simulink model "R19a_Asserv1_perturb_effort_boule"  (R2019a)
settings: Solver=ode15s  StartTime=0.0  StopTime=1  RelTol=1e-3  EnableMultiTasking=on
undefined symbols (not defined in the file): deg, kg, m, manette1_Défaut_sldprt, manette2_Défaut_sldprt, mm, N, rad, s, sigbuilder_block, STL, X, Y, Z
libraries: sm_lib x460, fl_lib x45, nesl_utility x23, simulink x3
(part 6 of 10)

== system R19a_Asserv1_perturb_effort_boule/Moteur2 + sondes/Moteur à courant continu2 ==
  note: Kv = 1.18e-1
  Frottement : fl_lib/Mechanical/Rotational Elements/Rotational Friction  brkwy_trq=2.43e-3 N*m  brkwy_vel=0.030296 rad/s  Col_trq=2.43e-3 N*m  visc_coef=2e-6 N*m/(rad/s)  w_specify=off  w_priority=High  w=0 rad/s  w_nominal_specify=off  w_nominal_unit=rad/s  w_nominal_value=1  t_specify=off  t_priority=High  t=0 N*m  t_nominal_specify=off  t_nominal_unit=N*m  t_nominal_value=1
  Inductance induit 35mH : fl_lib/Electrical/Electrical Elements/Inductor  l=35 mH  r=0 Ohm  g=1e-09 1/Ohm  i_specify=off  i_priority=High  i=0 A  i_nominal_specify=off  i_nominal_unit=A  i_nominal_value=1  v_specify=off  v_priority=High  v=0 V  v_nominal_specify=off  v_nominal_unit=V  v_nominal_value=1  i_L_specify=on  i_L_priority=High  i_L=0 A  i_L_nominal_specify=off  i_L_nominal_unit=A  i_L_nominal_value=1
  Inertie Je 10e-6 : fl_lib/Mechanical/Rotational Elements/Inertia  inertia=10.5e-6 kg*m^2  w_specify=on  w_priority=High  w=0 rad/s  w_nominal_specify=off  w_nominal_unit=rad/s  w_nominal_value=1  t_specify=off  t_priority=High  t=0 N*m  t_nominal_specify=off  t_nominal_unit=N*m  t_nominal_value=1
  Moteur parfait : fl_lib/Electrical/Electrical Elements/Rotational Electromechanical Converter  K=1.18e-1 V/(rad/s)  i_specify=off  i_priority=High  i=0 A  i_nominal_specify=off  i_nominal_unit=A  i_nominal_value=1  v_specify=off  v_priority=High  v=0 V  v_nominal_specify=off  v_nominal_unit=V  v_nominal_value=1  t_specify=off  t_priority=High  t=0 N*m  t_nominal_specify=off  t_nominal_unit=N*m  t_nominal_value=1  w_specify=off  w_priority=High  w=0 rad/s  w_nominal_specify=off  w_nominal_unit=rad/s  w_nominal_value=1
  Rinduit 38 Ohms : fl_lib/Electrical/Electrical Elements/Resistor  Tag=Factory Generic  R=38 Ohm  i_specify=off  i_priority=High  i=0 A  i_nominal_specify=off  i_nominal_unit=A  i_nominal_value=1  v_specify=off  v_priority=High  v=0 V  v_nominal_specify=off  v_nominal_unit=V  v_nominal_value=1
  V+ : PMIOPort  Side=Left
  R : PMIOPort  Port=2  Side=Right
  C : PMIOPort  Port=3  Side=Right
  V- : PMIOPort  Port=4  Side=Left
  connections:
  Moteur parfait/LConn1 -- Inductance induit 35mH/RConn1
  V-/RConn1 -- Moteur parfait/RConn1
  Rinduit 38 Ohms/LConn1 -- V+/RConn1
  Inductance induit 35mH/LConn1 -- Rinduit 38 Ohms/RConn1
  Frottement/LConn1 -- Moteur parfait/LConn2 -- Inertie Je 10e-6/LConn1 -- R/RConn1
  Frottement/RConn1 -- Moteur parfait/RConn2 -- C/RConn1

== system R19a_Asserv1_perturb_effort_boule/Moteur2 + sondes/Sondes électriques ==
  " Conv i" : nesl_utility/PS-Simulink Converter  PhysicalDomain=network_engine_domain  SubClassName=ps_output  LeftPortType=input  RightPortType=output  PseudoPeriodic=off  Frequencies=[]  Unit=1  AffineConversion=off
  " Conv v" : nesl_utility/PS-Simulink Converter  PhysicalDomain=network_engine_domain  SubClassName=ps_output  LeftPortType=input  RightPortType=output  PseudoPeriodic=off  Frequencies=[]  Unit=1  AffineConversion=off
  Bras2 : Scope  NumInputPorts=2
  Sonde_I : fl_lib/Electrical/Electrical Sensors/Current Sensor
  Sonde_U : fl_lib/Electrical/Electrical Sensors/Voltage Sensor
  Conn1 : PMIOPort  Side=Left
  Conn2 : PMIOPort  Port=2  Side=Right
  Conn3 : PMIOPort  Port=3  Side=Right
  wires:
  " Conv v"/1 -> [u]
  " Conv i"/1 -> [i]
  [u] -> Bras2/1  "Umoteur2"
  [i] -> Bras2/2  "Imoteur2"
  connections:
  Sonde_I/RConn1 -- " Conv i"/LConn1
  Sonde_U/RConn1 -- " Conv v"/LConn1
  Conn1/RConn1 -- Sonde_U/LConn1 -- Sonde_I/LConn1
  Conn2/RConn1 -- Sonde_I/RConn2
  Conn3/RConn1 -- Sonde_U/RConn2

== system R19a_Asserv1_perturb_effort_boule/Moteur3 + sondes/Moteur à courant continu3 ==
  note: Kv = 1.18e-1
  Frottement : fl_lib/Mechanical/Rotational Elements/Rotational Friction  brkwy_trq=2.43e-3 N*m  brkwy_vel=0.030296 rad/s  Col_trq=2.43e-3 N*m  visc_coef=2e-6 N*m/(rad/s)  w_specify=off  w_priority=High  w=0 rad/s  w_nominal_specify=off  w_nominal_unit=rad/s  w_nominal_value=1  t_specify=off  t_priority=High  t=0 N*m  t_nominal_specify=off  t_nominal_unit=N*m  t_nominal_value=1
  Inductance induit 35mH : fl_lib/Electrical/Electrical Elements/Inductor  l=35 mH  r=0 Ohm  g=1e-09 1/Ohm  i_specify=off  i_priority=High  i=0 A  i_nominal_specify=off  i_nominal_unit=A  i_nominal_value=1  v_specify=off  v_priority=High  v=0 V  v_nominal_specify=off  v_nominal_unit=V  v_nominal_value=1  i_L_specify=on  i_L_priority=High  i_L=0 A  i_L_nominal_specify=off  i_L_nominal_unit=A  i_L_nominal_value=1
  Inertie Je 10e-6 : fl_lib/Mechanical/Rotational Elements/Inertia  inertia=10.5e-6 kg*m^2  w_specify=on  w_priority=High  w=0 rad/s  w_nominal_specify=off  w_nominal_unit=rad/s  w_nominal_value=1  t_specify=off  t_priority=High  t=0 N*m  t_nominal_specify=off  t_nominal_unit=N*m  t_nominal_value=1
  Moteur parfait : fl_lib/Electrical/Electrical Elements/Rotational Electromechanical Converter  K=1.18e-1 V/(rad/s)  i_specify=off  i_priority=High  i=0 A  i_nominal_specify=off  i_nominal_unit=A  i_nominal_value=1  v_specify=off  v_priority=High  v=0 V  v_nominal_specify=off  v_nominal_unit=V  v_nominal_value=1  t_specify=off  t_priority=High  t=0 N*m  t_nominal_specify=off  t_nominal_unit=N*m  t_nominal_value=1  w_specify=off  w_priority=High  w=0 rad/s  w_nominal_specify=off  w_nominal_unit=rad/s  w_nominal_value=1
  Rinduit 38 Ohms : fl_lib/Electrical/Electrical Elements/Resistor  Tag=Factory Generic  R=38 Ohm  i_specify=off  i_priority=High  i=0 A  i_nominal_specify=off  i_nominal_unit=A  i_nominal_value=1  v_specify=off  v_priority=High  v=0 V  v_nominal_specify=off  v_nominal_unit=V  v_nominal_value=1
  V+ : PMIOPort  Side=Left
  R : PMIOPort  Port=2  Side=Right
  C : PMIOPort  Port=3  Side=Right
  V- : PMIOPort  Port=4  Side=Left
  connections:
  Moteur parfait/LConn1 -- Inductance induit 35mH/RConn1
  V-/RConn1 -- Moteur parfait/RConn1
  Rinduit 38 Ohms/LConn1 -- V+/RConn1
  Inductance induit 35mH/LConn1 -- Rinduit 38 Ohms/RConn1
  Frottement/LConn1 -- Moteur parfait/LConn2 -- Inertie Je 10e-6/LConn1 -- R/RConn1
  Frottement/RConn1 -- Moteur parfait/RConn2 -- C/RConn1

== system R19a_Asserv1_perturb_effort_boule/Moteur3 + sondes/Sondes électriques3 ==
  " Conv i" : nesl_utility/PS-Simulink Converter  PhysicalDomain=network_engine_domain  SubClassName=ps_output  LeftPortType=input  RightPortType=output  PseudoPeriodic=off  Frequencies=[]  Unit=1  AffineConversion=off
  " Conv v" : nesl_utility/PS-Simulink Converter  PhysicalDomain=network_engine_domain  SubClassName=ps_output  LeftPortType=input  RightPortType=output  PseudoPeriodic=off  Frequencies=[]  Unit=1  AffineConversion=off
  Bras3 : Scope  NumInputPorts=2
  Sonde_I : fl_lib/Electrical/Electrical Sensors/Current Sensor
  Sonde_U : fl_lib/Electrical/Electrical Sensors/Voltage Sensor
  Conn1 : PMIOPort  Side=Left
  Conn2 : PMIOPort  Port=2  Side=Right
  Conn3 : PMIOPort  Port=3  Side=Right
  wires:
  " Conv v"/1 -> [u]
  " Conv i"/1 -> [i]
  [u] -> Bras3/1  "Umoteur3"
  [i] -> Bras3/2  "Imoteur3"
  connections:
  Sonde_I/RConn1 -- " Conv i"/LConn1
  Sonde_U/RConn1 -- " Conv v"/LConn1
  Conn1/RConn1 -- Sonde_U/LConn1 -- Sonde_I/LConn1
  Conn2/RConn1 -- Sonde_I/RConn2
  Conn3/RConn1 -- Sonde_U/RConn2

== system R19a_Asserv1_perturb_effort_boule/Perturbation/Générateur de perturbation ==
  Demux : Demux  Tag=STV Demux  Outputs=1
  FromWs : FromWorkspace  Tag=STV FromWs  VariableName=tuvar  SampleTime=0
  Signal 1 : Outport  Tag=STV Outport
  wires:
  Demux/1 -> Signal 1/1
  FromWs/1 -> Demux/1

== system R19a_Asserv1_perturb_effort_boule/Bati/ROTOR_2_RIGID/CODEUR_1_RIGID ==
  ReferenceFrame : sm_lib/Frames and Transforms/Reference Frame
  Solid : sm_lib/Body Elements/Solid  InertiaType=Custom  Mass=0.0064318274490095598  MassUnits=kg  CenterOfMass=[0 6.0527709306807029 -0.1964144966449296]  CenterOfMassUnits=mm  MomentsOfInertia=[0.92812714377460337 1.2443807481520079 0.93469179577802664]  MomentsOfInertiaUnits=kg*mm^2  ProductsOfInertia=[0.0063987198741970201 0 0]  ProductsOfInertiaUnits=kg*mm^2  BasedOnType=Density  Density=1000  DensityUnits=kg/(m^3)  DoExposeReferenceFrame=on  SerializedFrames=<Frames/>  GraphicType=FromGeometry  MarkerShape=Sphere  MarkerSize=10  MarkerSizeUnits=m  GraphicVisPropType=SimpleVisualProperties  GraphicDiffuseColor=[0.2 1.0 0.2]  GraphicSpecularColor=[0.5 0.5 0.5 1.0]  GraphicAmbientColor=[0.15 0.15 0.15 1.0]  GraphicEmissiveColor=[0.0 0.0 0.0 1.0]  GraphicShininess=75  GraphicOpacity=1  GeometryShape=FromFile  RectangleSize=[1 1]  RectangleSizeUnits=m  BrickDimensions=[1 1 1]  BrickDimensionUnits=m  CylinderRadius=1  CylinderRadiusUnits=m  CylinderLength=1  CylinderLengthUnits=m  SphereRadius=1  SphereRadiusUnits=m  EllipsoidRadii=[1 1 1]  EllipsoidRadiiUnits=m  ExtrusionCrossSection=[1 1; -1 1; -1 -1; 1 -1]  ExtrusionCrossSectionUnits=m  ExtrusionLength=1  ExtrusionLengthUnits=m  PolygonNumSides=3  PolygonOuterRadius=1  PolygonOuterRadiusUnits=m  ExtGeomFileType=STL  ExtGeomFileName=\STL\CODEUR_Défaut_sldprt.STL  ExtGeomFileUnits=mm  RevolutionCrossSection=[1 1; 1 -1; 2 -1; 2 1]  RevolutionCrossSectionUnits=m  RevolutionExtent=Full  RevolutionAngle=180  RevolutionAngleUnits=deg
  F : PMIOPort  Side=Left
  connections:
  Solid/RConn1 -- ReferenceFrame/RConn1 -- F/RConn1

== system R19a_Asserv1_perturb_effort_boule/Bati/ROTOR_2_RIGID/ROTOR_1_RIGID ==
  ReferenceFrame : sm_lib/Frames and Transforms/Reference Frame
  Solid : sm_lib/Body Elements/Solid  InertiaType=Custom  Mass=0.07643998420030651  MassUnits=kg  CenterOfMass=[0 30.928341108151987 -0.0018262913863015125]  CenterOfMassUnits=mm  MomentsOfInertia=[14.640748377051393 9.6696912582654697 14.640902193857929]  MomentsOfInertiaUnits=kg*mm^2  ProductsOfInertia=[0.0065014820412302417 0 0]  ProductsOfInertiaUnits=kg*mm^2  BasedOnType=Density  Density=1000  DensityUnits=kg/(m^3)  DoExposeReferenceFrame=on  SerializedFrames=<Frames/>  GraphicType=FromGeometry  MarkerShape=Sphere  MarkerSize=10  MarkerSizeUnits=m  GraphicVisPropType=SimpleVisualProperties  GraphicDiffuseColor=[0.53725490196078429 0.34901960784313724 0.33725490196078434]  GraphicSpecularColor=[0.5 0.5 0.5 1.0]  GraphicAmbientColor=[0.15 0.15 0.15 1.0]  GraphicEmissiveColor=[0.0 0.0 0.0 1.0]  GraphicShininess=75  GraphicOpacity=1  GeometryShape=FromFile  RectangleSize=[1 1]  RectangleSizeUnits=m  BrickDimensions=[1 1 1]  BrickDimensionUnits=m  CylinderRadius=1  CylinderRadiusUnits=m  CylinderLength=1  CylinderLengthUnits=m  SphereRadius=1  SphereRadiusUnits=m  EllipsoidRadii=[1 1 1]  EllipsoidRadiiUnits=m  ExtrusionCrossSection=[1 1; -1 1; -1 -1; 1 -1]  ExtrusionCrossSectionUnits=m  ExtrusionLength=1  ExtrusionLengthUnits=m  PolygonNumSides=3  PolygonOuterRadius=1  PolygonOuterRadiusUnits=m  ExtGeomFileType=STL  ExtGeomFileName=\STL\ROTOR_Défaut_sldprt.STL  ExtGeomFileUnits=mm  RevolutionCrossSection=[1 1; 1 -1; 2 -1; 2 1]  RevolutionCrossSectionUnits=m  RevolutionExtent=Full  RevolutionAngle=180  RevolutionAngleUnits=deg
  F : PMIOPort  Side=Left
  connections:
  Solid/RConn1 -- ReferenceFrame/RConn1 -- F/RConn1

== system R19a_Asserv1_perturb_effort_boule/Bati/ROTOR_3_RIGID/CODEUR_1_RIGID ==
  ReferenceFrame : sm_lib/Frames and Transforms/Reference Frame
  Solid : sm_lib/Body Elements/Solid  InertiaType=Custom  Mass=0.0064318274490095598  MassUnits=kg  CenterOfMass=[0 6.0527709306807029 -0.1964144966449296]  CenterOfMassUnits=mm  MomentsOfInertia=[0.92812714377460337 1.2443807481520079 0.93469179577802664]  MomentsOfInertiaUnits=kg*mm^2  ProductsOfInertia=[0.0063987198741970201 0 0]  ProductsOfInertiaUnits=kg*mm^2  BasedOnType=Density  Density=1000  DensityUnits=kg/(m^3)  DoExposeReferenceFrame=on  SerializedFrames=<Frames/>  GraphicType=FromGeometry  MarkerShape=Sphere  MarkerSize=10  MarkerSizeUnits=m  GraphicVisPropType=SimpleVisualProperties  GraphicDiffuseColor=[0.792156862745098 0.81960784313725488 0.93333333333333335]  GraphicSpecularColor=[0.5 0.5 0.5 1.0]  GraphicAmbientColor=[0.15 0.15 0.15 1.0]  GraphicEmissiveColor=[0.0 0.0 0.0 1.0]  GraphicShininess=75  GraphicOpacity=1  GeometryShape=FromFile  RectangleSize=[1 1]  RectangleSizeUnits=m  BrickDimensions=[1 1 1]  BrickDimensionUnits=m  CylinderRadius=1  CylinderRadiusUnits=m  CylinderLength=1  CylinderLengthUnits=m  SphereRadius=1  SphereRadiusUnits=m  EllipsoidRadii=[1 1 1]  EllipsoidRadiiUnits=m  ExtrusionCrossSection=[1 1; -1 1; -1 -1; 1 -1]  ExtrusionCrossSectionUnits=m  ExtrusionLength=1  ExtrusionLengthUnits=m  PolygonNumSides=3  PolygonOuterRadius=1  PolygonOuterRadiusUnits=m  ExtGeomFileType=STL  ExtGeomFileName=\STL\CODEUR_Défaut_sldprt.STL  ExtGeomFileUnits=mm  RevolutionCrossSection=[1 1; 1 -1; 2 -1; 2 1]  RevolutionCrossSectionUnits=m  RevolutionExtent=Full  RevolutionAngle=180  RevolutionAngleUnits=deg
  F : PMIOPort  Side=Left
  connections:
  Solid/RConn1 -- ReferenceFrame/RConn1 -- F/RConn1

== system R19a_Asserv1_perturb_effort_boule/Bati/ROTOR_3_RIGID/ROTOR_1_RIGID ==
  ReferenceFrame : sm_lib/Frames and Transforms/Reference Frame
  Solid : sm_lib/Body Elements/Solid  InertiaType=Custom  Mass=0.07643998420030651  MassUnits=kg  CenterOfMass=[0 30.928341108151987 -0.0018262913863015125]  CenterOfMassUnits=mm  MomentsOfInertia=[14.640748377051393 9.6696912582654697 14.640902193857929]  MomentsOfInertiaUnits=kg*mm^2  ProductsOfInertia=[0.0065014820412302417 0 0]  ProductsOfInertiaUnits=kg*mm^2  BasedOnType=Density  Density=1000  DensityUnits=kg/(m^3)  DoExposeReferenceFrame=on  SerializedFrames=<Frames/>  GraphicType=FromGeometry  MarkerShape=Sphere  MarkerSize=10  MarkerSizeUnits=m  GraphicVisPropType=SimpleVisualProperties  GraphicDiffuseColor=[0.53725490196078429 0.34901960784313724 0.33725490196078434]  GraphicSpecularColor=[0.5 0.5 0.5 1.0]  GraphicAmbientColor=[0.15 0.15 0.15 1.0]  GraphicEmissiveColor=[0.0 0.0 0.0 1.0]  GraphicShininess=75  GraphicOpacity=1  GeometryShape=FromFile  RectangleSize=[1 1]  RectangleSizeUnits=m  BrickDimensions=[1 1 1]  BrickDimensionUnits=m  CylinderRadius=1  CylinderRadiusUnits=m  CylinderLength=1  CylinderLengthUnits=m  SphereRadius=1  SphereRadiusUnits=m  EllipsoidRadii=[1 1 1]  EllipsoidRadiiUnits=m  ExtrusionCrossSection=[1 1; -1 1; -1 -1; 1 -1]  ExtrusionCrossSectionUnits=m  ExtrusionLength=1  ExtrusionLengthUnits=m  PolygonNumSides=3  PolygonOuterRadius=1  PolygonOuterRadiusUnits=m  ExtGeomFileType=STL  ExtGeomFileName=\STL\ROTOR_Défaut_sldprt.STL  ExtGeomFileUnits=mm  RevolutionCrossSection=[1 1; 1 -1; 2 -1; 2 1]  RevolutionCrossSectionUnits=m  RevolutionExtent=Full  RevolutionAngle=180  RevolutionAngleUnits=deg
  F : PMIOPort  Side=Left
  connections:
  Solid/RConn1 -- ReferenceFrame/RConn1 -- F/RConn1

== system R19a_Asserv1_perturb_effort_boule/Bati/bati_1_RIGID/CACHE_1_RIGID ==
  ReferenceFrame : sm_lib/Frames and Transforms/Reference Frame
  Solid : sm_lib/Body Elements/Solid  InertiaType=Custom  Mass=0.011182198960412355  MassUnits=kg  CenterOfMass=[4.3076392714328797 208.54208665729635 7.8822671814956502]  CenterOfMassUnits=mm  MomentsOfInertia=[9.7659613803690544 11.857978985199471 3.5448360594417863]  MomentsOfInertiaUnits=kg*mm^2  ProductsOfInertia=[-0.087124917777044883 -0.069374532976861802 0.10473407202046144]  ProductsOfInertiaUnits=kg*mm^2  BasedOnType=Density  Density=1000  DensityUnits=kg/(m^3)  DoExposeReferenceFrame=on  SerializedFrames=<Frames/>  GraphicType=FromGeometry  MarkerShape=Sphere  MarkerSize=10  MarkerSizeUnits=m  GraphicVisPropType=SimpleVisualProperties  GraphicDiffuseColor=[0.75294117647058822 0.75294117647058822 0.75294117647058822]  GraphicSpecularColor=[0.5 0.5 0.5 1.0]  GraphicAmbientColor=[0.15 0.15 0.15 1.0]  GraphicEmissiveColor=[0.0 0.0 0.0 1.0]  GraphicShininess=75  GraphicOpacity=1  GeometryShape=FromFile  RectangleSize=[1 1]  RectangleSizeUnits=m  BrickDimensions=[1 1 1]  BrickDimensionUnits=m  CylinderRadius=1  CylinderRadiusUnits=m  CylinderLength=1  CylinderLengthUnits=m  SphereRadius=1  SphereRadiusUnits=m  EllipsoidRadii=[1 1 1]  EllipsoidRadiiUnits=m  ExtrusionCrossSection=[1 1; -1 1; -1 -1; 1 -1]  ExtrusionCrossSectionUnits=m  ExtrusionLength=1  ExtrusionLengthUnits=m  PolygonNumSides=3  PolygonOuterRadius=1  PolygonOuterRadiusUnits=m  ExtGeomFileType=STL  ExtGeomFileName=\STL\CACHE_Défaut_sldprt.STL  ExtGeomFileUnits=mm  RevolutionCrossSection=[1 1; 1 -1; 2 -1; 2 1]  RevolutionCrossSectionUnits=m  RevolutionExtent=Full  RevolutionAngle=180  RevolutionAngleUnits=deg
  F : PMIOPort  Side=Left
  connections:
  Solid/RConn1 -- ReferenceFrame/RConn1 -- F/RConn1

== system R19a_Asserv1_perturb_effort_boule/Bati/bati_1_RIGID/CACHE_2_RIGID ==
  ReferenceFrame : sm_lib/Frames and Transforms/Reference Frame
  Solid : sm_lib/Body Elements/Solid  InertiaType=Custom  Mass=0.011182198960412355  MassUnits=kg  CenterOfMass=[4.3076392714328797 208.54208665729635 7.8822671814956502]  CenterOfMassUnits=mm  MomentsOfInertia=[9.7659613803690544 11.857978985199471 3.5448360594417863]  MomentsOfInertiaUnits=kg*mm^2  ProductsOfInertia=[-0.087124917777044883 -0.069374532976861802 0.10473407202046144]  ProductsOfInertiaUnits=kg*mm^2  BasedOnType=Density  Density=1000  DensityUnits=kg/(m^3)  DoExposeReferenceFrame=on  SerializedFrames=<Frames/>  GraphicType=FromGeometry  MarkerShape=Sphere  MarkerSize=10  MarkerSizeUnits=m  GraphicVisPropType=SimpleVisualProperties  GraphicDiffuseColor=[0.75294117647058822 0.75294117647058822 0.75294117647058822]  GraphicSpecularColor=[0.5 0.5 0.5 1.0]  GraphicAmbientColor=[0.15 0.15 0.15 1.0]  GraphicEmissiveColor=[0.0 0.0 0.0 1.0]  GraphicShininess=75  GraphicOpacity=1  GeometryShape=FromFile  RectangleSize=[1 1]  RectangleSizeUnits=m  BrickDimensions=[1 1 1]  BrickDimensionUnits=m  CylinderRadius=1  CylinderRadiusUnits=m  CylinderLength=1  CylinderLengthUnits=m  SphereRadius=1  SphereRadiusUnits=m  EllipsoidRadii=[1 1 1]  EllipsoidRadiiUnits=m  ExtrusionCrossSection=[1 1; -1 1; -1 -1; 1 -1]  ExtrusionCrossSectionUnits=m  ExtrusionLength=1  ExtrusionLengthUnits=m  PolygonNumSides=3  PolygonOuterRadius=1  PolygonOuterRadiusUnits=m  ExtGeomFileType=STL  ExtGeomFileName=\STL\CACHE_Défaut_sldprt.STL  ExtGeomFileUnits=mm  RevolutionCrossSection=[1 1; 1 -1; 2 -1; 2 1]  RevolutionCrossSectionUnits=m  RevolutionExtent=Full  RevolutionAngle=180  RevolutionAngleUnits=deg
  F : PMIOPort  Side=Left
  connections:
  Solid/RConn1 -- ReferenceFrame/RConn1 -- F/RConn1

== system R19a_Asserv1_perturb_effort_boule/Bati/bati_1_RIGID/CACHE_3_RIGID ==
  ReferenceFrame : sm_lib/Frames and Transforms/Reference Frame
  Solid : sm_lib/Body Elements/Solid  InertiaType=Custom  Mass=0.011182198960412355  MassUnits=kg  CenterOfMass=[4.3076392714328797 208.54208665729635 7.8822671814956502]  CenterOfMassUnits=mm  MomentsOfInertia=[9.7659613803690544 11.857978985199471 3.5448360594417863]  MomentsOfInertiaUnits=kg*mm^2  ProductsOfInertia=[-0.087124917777044883 -0.069374532976861802 0.10473407202046144]  ProductsOfInertiaUnits=kg*mm^2  BasedOnType=Density  Density=1000  DensityUnits=kg/(m^3)  DoExposeReferenceFrame=on  SerializedFrames=<Frames/>  GraphicType=FromGeometry  MarkerShape=Sphere  MarkerSize=10  MarkerSizeUnits=m  GraphicVisPropType=SimpleVisualProperties  GraphicDiffuseColor=[0.75294117647058822 0.75294117647058822 0.75294117647058822]  GraphicSpecularColor=[0.5 0.5 0.5 1.0]  GraphicAmbientColor=[0.15 0.15 0.15 1.0]  GraphicEmissiveColor=[0.0 0.0 0.0 1.0]  GraphicShininess=75  GraphicOpacity=1  GeometryShape=FromFile  RectangleSize=[1 1]  RectangleSizeUnits=m  BrickDimensions=[1 1 1]  BrickDimensionUnits=m  CylinderRadius=1  CylinderRadiusUnits=m  CylinderLength=1  CylinderLengthUnits=m  SphereRadius=1  SphereRadiusUnits=m  EllipsoidRadii=[1 1 1]  EllipsoidRadiiUnits=m  ExtrusionCrossSection=[1 1; -1 1; -1 -1; 1 -1]  ExtrusionCrossSectionUnits=m  ExtrusionLength=1  ExtrusionLengthUnits=m  PolygonNumSides=3  PolygonOuterRadius=1  PolygonOuterRadiusUnits=m  ExtGeomFileType=STL  ExtGeomFileName=\STL\CACHE_Défaut_sldprt.STL  ExtGeomFileUnits=mm  RevolutionCrossSection=[1 1; 1 -1; 2 -1; 2 1]  RevolutionCrossSectionUnits=m  RevolutionExtent=Full  RevolutionAngle=180  RevolutionAngleUnits=deg
  F : PMIOPort  Side=Left
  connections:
  Solid/RConn1 -- ReferenceFrame/RConn1 -- F/RConn1

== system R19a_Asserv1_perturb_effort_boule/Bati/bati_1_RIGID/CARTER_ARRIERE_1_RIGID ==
  ReferenceFrame : sm_lib/Frames and Transforms/Reference Frame
  Solid : sm_lib/Body Elements/Solid  InertiaType=Custom  Mass=0.12081050845213158  MassUnits=kg  CenterOfMass=[0.027688933623677491 107.2258121438302 -1.1182869436416025]  CenterOfMassUnits=mm  MomentsOfInertia=[436.20873458136924 359.38976174708495 770.46596034318191]  MomentsOfInertiaUnits=kg*mm^2  ProductsOfInertia=[18.068269630416292 -0.016904145152124985 0.032703140147255623]  ProductsOfInertiaUnits=kg*mm^2  BasedOnType=Density  Density=1000  DensityUnits=kg/(m^3)  DoExposeReferenceFrame=on  SerializedFrames=<Frames/>  GraphicType=FromGeometry  MarkerShape=Sphere  MarkerSize=10  MarkerSizeUnits=m  GraphicVisPropType=SimpleVisualProperties  GraphicDiffuseColor=[1 1 1]  GraphicSpecularColor=[0.5 0.5 0.5 1.0]  GraphicAmbientColor=[0.15 0.15 0.15 1.0]  GraphicEmissiveColor=[0.0 0.0 0.0 1.0]  GraphicShininess=75  GraphicOpacity=1  GeometryShape=FromFile  RectangleSize=[1 1]  RectangleSizeUnits=m  BrickDimensions=[1 1 1]  BrickDimensionUnits=m  CylinderRadius=1  CylinderRadiusUnits=m  CylinderLength=1  CylinderLengthUnits=m  SphereRadius=1  SphereRadiusUnits=m  EllipsoidRadii=[1 1 1]  EllipsoidRadiiUnits=m  ExtrusionCrossSection=[1 1; -1 1; -1 -1; 1 -1]  ExtrusionCrossSectionUnits=m  ExtrusionLength=1  ExtrusionLengthUnits=m  PolygonNumSides=3  PolygonOuterRadius=1  PolygonOuterRadiusUnits=m  ExtGeomFileType=STL  ExtGeomFileName=\STL\CARTER ARRIERE_Défaut_sldprt.STL  ExtGeomFileUnits=mm  RevolutionCrossSection=[1 1; 1 -1; 2 -1; 2 1]  RevolutionCrossSectionUnits=m  RevolutionExtent=Full  RevolutionAngle=180  RevolutionAngleUnits=deg
  F : PMIOPort  Side=Left
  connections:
  Solid/RConn1 -- ReferenceFrame/RConn1 -- F/RConn1

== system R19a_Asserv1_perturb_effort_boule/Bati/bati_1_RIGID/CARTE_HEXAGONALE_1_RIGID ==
  ReferenceFrame : sm_lib/Frames and Transforms/Reference Frame
  Solid : sm_lib/Body Elements/Solid  InertiaType=Custom  Mass=0.026994433881078982  MassUnits=kg  CenterOfMass=[-1.609455224288012 -0.90517012664311758 2.5720012204185174]  CenterOfMassUnits=mm  MomentsOfInertia=[28.923221067904205 24.898136547803855 53.038824077161053]  MomentsOfInertiaUnits=kg*mm^2  ProductsOfInertia=[0.34251255903735656 0.14956628541838315 1.4697500359655211]  ProductsOfInertiaUnits=kg*mm^2  BasedOnType=Density  Density=1000  DensityUnits=kg/(m^3)  DoExposeReferenceFrame=on  SerializedFrames=<Frames/>  GraphicType=FromGeometry  MarkerShape=Sphere  MarkerSize=10  MarkerSizeUnits=m  GraphicVisPropType=SimpleVisualProperties  GraphicDiffuseColor=[0 0.50196078431372548 0]  GraphicSpecularColor=[0.5 0.5 0.5 1.0]  GraphicAmbientColor=[0.15 0.15 0.15 1.0]  GraphicEmissiveColor=[0.0 0.0 0.0 1.0]  GraphicShininess=75  GraphicOpacity=1  GeometryShape=FromFile  RectangleSize=[1 1]  RectangleSizeUnits=m  BrickDimensions=[1 1 1]  BrickDimensionUnits=m  CylinderRadius=1  CylinderRadiusUnits=m  CylinderLength=1  CylinderLengthUnits=m  SphereRadius=1  SphereRadiusUnits=m  EllipsoidRadii=[1 1 1]  EllipsoidRadiiUnits=m  ExtrusionCrossSection=[1 1; -1 1; -1 -1; 1 -1]  ExtrusionCrossSectionUnits=m  ExtrusionLength=1  ExtrusionLengthUnits=m  PolygonNumSides=3  PolygonOuterRadius=1  PolygonOuterRadiusUnits=m  ExtGeomFileType=STL  ExtGeomFileName=\STL\CARTE HEXAGONALE_Défaut_sldprt.STL  ExtGeomFileUnits=mm  RevolutionCrossSection=[1 1; 1 -1; 2 -1; 2 1]  RevolutionCrossSectionUnits=m  RevolutionExtent=Full  RevolutionAngle=180  RevolutionAngleUnits=deg
  F : PMIOPort  Side=Left
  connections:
  Solid/RConn1 -- ReferenceFrame/RConn1 -- F/RConn1

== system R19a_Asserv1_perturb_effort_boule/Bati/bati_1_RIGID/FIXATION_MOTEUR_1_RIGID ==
  ReferenceFrame : sm_lib/Frames and Transforms/Reference Frame
  Solid : sm_lib/Body Elements/Solid  InertiaType=Custom  Mass=0.00025251914881442344  MassUnits=kg  CenterOfMass=[0 10.662239702438894 0]  CenterOfMassUnits=mm  MomentsOfInertia=[0.012730499644358427 0.059038940284933263 0.070228178640671796]  MomentsOfInertiaUnits=kg*mm^2  ProductsOfInertia=[0 0 0]  ProductsOfInertiaUnits=kg*mm^2  BasedOnType=Density  Density=1000  DensityUnits=kg/(m^3)  DoExposeReferenceFrame=on  SerializedFrames=<Frames/>  GraphicType=FromGeometry  MarkerShape=Sphere  MarkerSize=10  MarkerSizeUnits=m  GraphicVisPropType=SimpleVisualProperties  GraphicDiffuseColor=[0.792156862745098 0.81960784313725488 0.93333333333333335]  GraphicSpecularColor=[0.5 0.5 0.5 1.0]  GraphicAmbientColor=[0.15 0.15 0.15 1.0]  GraphicEmissiveColor=[0.0 0.0 0.0 1.0]  GraphicShininess=75  GraphicOpacity=1  GeometryShape=FromFile  RectangleSize=[1 1]  RectangleSizeUnits=m  BrickDimensions=[1 1 1]  BrickDimensionUnits=m  CylinderRadius=1  CylinderRadiusUnits=m  CylinderLength=1  CylinderLengthUnits=m  SphereRadius=1  SphereRadiusUnits=m  EllipsoidRadii=[1 1 1]  EllipsoidRadiiUnits=m  ExtrusionCrossSection=[1 1; -1 1; -1 -1; 1 -1]  ExtrusionCrossSectionUnits=m  ExtrusionLength=1  ExtrusionLengthUnits=m  PolygonNumSides=3  PolygonOuterRadius=1  PolygonOuterRadiusUnits=m  ExtGeomFileType=STL  ExtGeomFileName=\STL\FIXATION MOTEUR_Défaut_sldprt.STL  ExtGeomFileUnits=mm  RevolutionCrossSection=[1 1; 1 -1; 2 -1; 2 1]  RevolutionCrossSectionUnits=m  RevolutionExtent=Full  RevolutionAngle=180  RevolutionAngleUnits=deg
  F : PMIOPort  Side=Left
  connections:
  Solid/RConn1 -- ReferenceFrame/RConn1 -- F/RConn1

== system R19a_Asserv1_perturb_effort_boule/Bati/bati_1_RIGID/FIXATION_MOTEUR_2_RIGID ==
  ReferenceFrame : sm_lib/Frames and Transforms/Reference Frame
  Solid : sm_lib/Body Elements/Solid  InertiaType=Custom  Mass=0.00025251914881442344  MassUnits=kg  CenterOfMass=[0 10.662239702438894 0]  CenterOfMassUnits=mm  MomentsOfInertia=[0.012730499644358427 0.059038940284933263 0.070228178640671796]  MomentsOfInertiaUnits=kg*mm^2  ProductsOfInertia=[0 0 0]  ProductsOfInertiaUnits=kg*mm^2  BasedOnType=Density  Density=1000  DensityUnits=kg/(m^3)  DoExposeReferenceFrame=on  SerializedFrames=<Frames/>  GraphicType=FromGeometry  MarkerShape=Sphere  MarkerSize=10  MarkerSizeUnits=m  GraphicVisPropType=SimpleVisualProperties  GraphicDiffuseColor=[0.792156862745098 0.81960784313725488 0.93333333333333335]  GraphicSpecularColor=[0.5 0.5 0.5 1.0]  GraphicAmbientColor=[0.15 0.15 0.15 1.0]  GraphicEmissiveColor=[0.0 0.0 0.0 1.0]  GraphicShininess=75  GraphicOpacity=1  GeometryShape=FromFile  RectangleSize=[1 1]  RectangleSizeUnits=m  BrickDimensions=[1 1 1]  BrickDimensionUnits=m  CylinderRadius=1  CylinderRadiusUnits=m  CylinderLength=1  CylinderLengthUnits=m  SphereRadius=1  SphereRadiusUnits=m  EllipsoidRadii=[1 1 1]  EllipsoidRadiiUnits=m  ExtrusionCrossSection=[1 1; -1 1; -1 -1; 1 -1]  ExtrusionCrossSectionUnits=m  ExtrusionLength=1  ExtrusionLengthUnits=m  PolygonNumSides=3  PolygonOuterRadius=1  PolygonOuterRadiusUnits=m  ExtGeomFileType=STL  ExtGeomFileName=\STL\FIXATION MOTEUR_Défaut_sldprt.STL  ExtGeomFileUnits=mm  RevolutionCrossSection=[1 1; 1 -1; 2 -1; 2 1]  RevolutionCrossSectionUnits=m  RevolutionExtent=Full  RevolutionAngle=180  RevolutionAngleUnits=deg
  F : PMIOPort  Side=Left
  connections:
  Solid/RConn1 -- ReferenceFrame/RConn1 -- F/RConn1

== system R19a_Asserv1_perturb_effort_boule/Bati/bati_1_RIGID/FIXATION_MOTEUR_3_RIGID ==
  ReferenceFrame : sm_lib/Frames and Transforms/Reference Frame
  Solid : sm_lib/Body Elements/Solid  InertiaType=Custom  Mass=0.00025251914881442344  MassUnits=kg  CenterOfMass=[0 10.662239702438894 0]  CenterOfMassUnits=mm  MomentsOfInertia=[0.012730499644358427 0.059038940284933263 0.070228178640671796]  MomentsOfInertiaUnits=kg*mm^2  ProductsOfInertia=[0 0 0]  ProductsOfInertiaUnits=kg*mm^2  BasedOnType=Density  Density=1000  DensityUnits=kg/(m^3)  DoExposeReferenceFrame=on  SerializedFrames=<Frames/>  GraphicType=FromGeometry  MarkerShape=Sphere  MarkerSize=10  MarkerSizeUnits=m  GraphicVisPropType=SimpleVisualProperties  GraphicDiffuseColor=[0.792156862745098 0.81960784313725488 0.93333333333333335]  GraphicSpecularColor=[0.5 0.5 0.5 1.0]  GraphicAmbientColor=[0.15 0.15 0.15 1.0]  GraphicEmissiveColor=[0.0 0.0 0.0 1.0]  GraphicShininess=75  GraphicOpacity=1  GeometryShape=FromFile  RectangleSize=[1 1]  RectangleSizeUnits=m  BrickDimensions=[1 1 1]  BrickDimensionUnits=m  CylinderRadius=1  CylinderRadiusUnits=m  CylinderLength=1  CylinderLengthUnits=m  SphereRadius=1  SphereRadiusUnits=m  EllipsoidRadii=[1 1 1]  EllipsoidRadiiUnits=m  ExtrusionCrossSection=[1 1; -1 1; -1 -1; 1 -1]  ExtrusionCrossSectionUnits=m  ExtrusionLength=1  ExtrusionLengthUnits=m  PolygonNumSides=3  PolygonOuterRadius=1  PolygonOuterRadiusUnits=m  ExtGeomFileType=STL  ExtGeomFileName=\STL\FIXATION MOTEUR_Défaut_sldprt.STL  ExtGeomFileUnits=mm  RevolutionCrossSection=[1 1; 1 -1; 2 -1; 2 1]  RevolutionCrossSectionUnits=m  RevolutionExtent=Full  RevolutionAngle=180  RevolutionAngleUnits=deg
  F : PMIOPort  Side=Left
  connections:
  Solid/RConn1 -- ReferenceFrame/RConn1 -- F/RConn1

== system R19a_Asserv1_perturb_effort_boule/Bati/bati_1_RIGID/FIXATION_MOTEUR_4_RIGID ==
  ReferenceFrame : sm_lib/Frames and Transforms/Reference Frame
  Solid : sm_lib/Body Elements/Solid  InertiaType=Custom  Mass=0.00025251914881442344  MassUnits=kg  CenterOfMass=[0 10.662239702438894 0]  CenterOfMassUnits=mm  MomentsOfInertia=[0.012730499644358427 0.059038940284933263 0.070228178640671796]  MomentsOfInertiaUnits=kg*mm^2  ProductsOfInertia=[0 0 0]  ProductsOfInertiaUnits=kg*mm^2  BasedOnType=Density  Density=1000  DensityUnits=kg/(m^3)  DoExposeReferenceFrame=on  SerializedFrames=<Frames/>  GraphicType=FromGeometry  MarkerShape=Sphere  MarkerSize=10  MarkerSizeUnits=m  GraphicVisPropType=SimpleVisualProperties  GraphicDiffuseColor=[0.792156862745098 0.81960784313725488 0.93333333333333335]  GraphicSpecularColor=[0.5 0.5 0.5 1.0]  GraphicAmbientColor=[0.15 0.15 0.15 1.0]  GraphicEmissiveColor=[0.0 0.0 0.0 1.0]  GraphicShininess=75  GraphicOpacity=1  GeometryShape=FromFile  RectangleSize=[1 1]  RectangleSizeUnits=m  BrickDimensions=[1 1 1]  BrickDimensionUnits=m  CylinderRadius=1  CylinderRadiusUnits=m  CylinderLength=1  CylinderLengthUnits=m  SphereRadius=1  SphereRadiusUnits=m  EllipsoidRadii=[1 1 1]  EllipsoidRadiiUnits=m  ExtrusionCrossSection=[1 1; -1 1; -1 -1; 1 -1]  ExtrusionCrossSectionUnits=m  ExtrusionLength=1  ExtrusionLengthUnits=m  PolygonNumSides=3  PolygonOuterRadius=1  PolygonOuterRadiusUnits=m  ExtGeomFileType=STL  ExtGeomFileName=\STL\FIXATION MOTEUR_Défaut_sldprt.STL  ExtGeomFileUnits=mm  RevolutionCrossSection=[1 1; 1 -1; 2 -1; 2 1]  RevolutionCrossSectionUnits=m  RevolutionExtent=Full  RevolutionAngle=180  RevolutionAngleUnits=deg
  F : PMIOPort  Side=Left
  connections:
  Solid/RConn1 -- ReferenceFrame/RConn1 -- F/RConn1

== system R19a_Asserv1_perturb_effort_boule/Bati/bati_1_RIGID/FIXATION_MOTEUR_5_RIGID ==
  ReferenceFrame : sm_lib/Frames and Transforms/Reference Frame
  Solid : sm_lib/Body Elements/Solid  InertiaType=Custom  Mass=0.00025251914881442344  MassUnits=kg  CenterOfMass=[0 10.662239702438894 0]  CenterOfMassUnits=mm  MomentsOfInertia=[0.012730499644358427 0.059038940284933263 0.070228178640671796]  MomentsOfInertiaUnits=kg*mm^2  ProductsOfInertia=[0 0 0]  ProductsOfInertiaUnits=kg*mm^2  BasedOnType=Density  Density=1000  DensityUnits=kg/(m^3)  DoExposeReferenceFrame=on  SerializedFrames=<Frames/>  GraphicType=FromGeometry  MarkerShape=Sphere  MarkerSize=10  MarkerSizeUnits=m  GraphicVisPropType=SimpleVisualProperties  GraphicDiffuseColor=[0.792156862745098 0.81960784313725488 0.93333333333333335]  GraphicSpecularColor=[0.5 0.5 0.5 1.0]  GraphicAmbientColor=[0.15 0.15 0.15 1.0]  GraphicEmissiveColor=[0.0 0.0 0.0 1.0]  GraphicShininess=75  GraphicOpacity=1  GeometryShape=FromFile  RectangleSize=[1 1]  RectangleSizeUnits=m  BrickDimensions=[1 1 1]  BrickDimensionUnits=m  CylinderRadius=1  CylinderRadiusUnits=m  CylinderLength=1  CylinderLengthUnits=m  SphereRadius=1  SphereRadiusUnits=m  EllipsoidRadii=[1 1 1]  EllipsoidRadiiUnits=m  ExtrusionCrossSection=[1 1; -1 1; -1 -1; 1 -1]  ExtrusionCrossSectionUnits=m  ExtrusionLength=1  ExtrusionLengthUnits=m  PolygonNumSides=3  PolygonOuterRadius=1  PolygonOuterRadiusUnits=m  ExtGeomFileType=STL  ExtGeomFileName=\STL\FIXATION MOTEUR_Défaut_sldprt.STL  ExtGeomFileUnits=mm  RevolutionCrossSection=[1 1; 1 -1; 2 -1; 2 1]  RevolutionCrossSectionUnits=m  RevolutionExtent=Full  RevolutionAngle=180  RevolutionAngleUnits=deg
  F : PMIOPort  Side=Left
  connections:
  Solid/RConn1 -- ReferenceFrame/RConn1 -- F/RConn1

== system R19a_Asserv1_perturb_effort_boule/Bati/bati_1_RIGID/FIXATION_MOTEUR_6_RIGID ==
  ReferenceFrame : sm_lib/Frames and Transforms/Reference Frame
  Solid : sm_lib/Body Elements/Solid  InertiaType=Custom  Mass=0.00025251914881442344  MassUnits=kg  CenterOfMass=[0 10.662239702438894 0]  CenterOfMassUnits=mm  MomentsOfInertia=[0.012730499644358427 0.059038940284933263 0.070228178640671796]  MomentsOfInertiaUnits=kg*mm^2  ProductsOfInertia=[0 0 0]  ProductsOfInertiaUnits=kg*mm^2  BasedOnType=Density  Density=1000  DensityUnits=kg/(m^3)  DoExposeReferenceFrame=on  SerializedFrames=<Frames/>  GraphicType=FromGeometry  MarkerShape=Sphere  MarkerSize=10  MarkerSizeUnits=m  GraphicVisPropType=SimpleVisualProperties  GraphicDiffuseColor=[0.792156862745098 0.81960784313725488 0.93333333333333335]  GraphicSpecularColor=[0.5 0.5 0.5 1.0]  GraphicAmbientColor=[0.15 0.15 0.15 1.0]  GraphicEmissiveColor=[0.0 0.0 0.0 1.0]  GraphicShininess=75  GraphicOpacity=1  GeometryShape=FromFile  RectangleSize=[1 1]  RectangleSizeUnits=m  BrickDimensions=[1 1 1]  BrickDimensionUnits=m  CylinderRadius=1  CylinderRadiusUnits=m  CylinderLength=1  CylinderLengthUnits=m  SphereRadius=1  SphereRadiusUnits=m  EllipsoidRadii=[1 1 1]  EllipsoidRadiiUnits=m  ExtrusionCrossSection=[1 1; -1 1; -1 -1; 1 -1]  ExtrusionCrossSectionUnits=m  ExtrusionLength=1  ExtrusionLengthUnits=m  PolygonNumSides=3  PolygonOuterRadius=1  PolygonOuterRadiusUnits=m  ExtGeomFileType=STL  ExtGeomFileName=\STL\FIXATION MOTEUR_Défaut_sldprt.STL  ExtGeomFileUnits=mm  RevolutionCrossSection=[1 1; 1 -1; 2 -1; 2 1]  RevolutionCrossSectionUnits=m  RevolutionExtent=Full  RevolutionAngle=180  RevolutionAngleUnits=deg
  F : PMIOPort  Side=Left
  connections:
  Solid/RConn1 -- ReferenceFrame/RConn1 -- F/RConn1

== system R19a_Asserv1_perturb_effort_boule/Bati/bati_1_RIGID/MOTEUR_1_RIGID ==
  ReferenceFrame : sm_lib/Frames and Transforms/Reference Frame
  Solid : sm_lib/Body Elements/Solid  InertiaType=Custom  Mass=0.064287172119754279  MassUnits=kg  CenterOfMass=[0 32.927342518193171 0]  CenterOfMassUnits=mm  MomentsOfInertia=[23.361167142247837 11.499741081133124 23.353822804254591]  MomentsOfInertiaUnits=kg*mm^2  ProductsOfInertia=[0 0 0]  ProductsOfInertiaUnits=kg*mm^2  BasedOnType=Density  Density=1000  DensityUnits=kg/(m^3)  DoExposeReferenceFrame=on  SerializedFrames=<Frames/>  GraphicType=FromGeometry  MarkerShape=Sphere  MarkerSize=10  MarkerSizeUnits=m  GraphicVisPropType=SimpleVisualProperties  GraphicDiffuseColor=[0.792156862745098 0.81960784313725488 0.93333333333333335]  GraphicSpecularColor=[0.5 0.5 0.5 1.0]  GraphicAmbientColor=[0.15 0.15 0.15 1.0]  GraphicEmissiveColor=[0.0 0.0 0.0 1.0]  GraphicShininess=75  GraphicOpacity=1  GeometryShape=FromFile  RectangleSize=[1 1]  RectangleSizeUnits=m  BrickDimensions=[1 1 1]  BrickDimensionUnits=m  CylinderRadius=1  CylinderRadiusUnits=m  CylinderLength=1  CylinderLengthUnits=m  SphereRadius=1  SphereRadiusUnits=m  EllipsoidRadii=[1 1 1]  EllipsoidRadiiUnits=m  ExtrusionCrossSection=[1 1; -1 1; -1 -1; 1 -1]  ExtrusionCrossSectionUnits=m  ExtrusionLength=1  ExtrusionLengthUnits=m  PolygonNumSides=3  PolygonOuterRadius=1  PolygonOuterRadiusUnits=m  ExtGeomFileType=STL  ExtGeomFileName=\STL\MOTEUR_Défaut_sldprt.STL  ExtGeomFileUnits=mm  RevolutionCrossSection=[1 1; 1 -1; 2 -1; 2 1]  RevolutionCrossSectionUnits=m  RevolutionExtent=Full  RevolutionAngle=180  RevolutionAngleUnits=deg
  F : PMIOPort  Side=Left
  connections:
  Solid/RConn1 -- ReferenceFrame/RConn1 -- F/RConn1

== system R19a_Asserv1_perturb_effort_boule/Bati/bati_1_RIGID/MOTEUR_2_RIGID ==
  ReferenceFrame : sm_lib/Frames and Transforms/Reference Frame
  Solid : sm_lib/Body Elements/Solid  InertiaType=Custom  Mass=0.064287172119754279  MassUnits=kg  CenterOfMass=[0 32.927342518193171 0]  CenterOfMassUnits=mm  MomentsOfInertia=[23.361167142247837 11.499741081133124 23.353822804254591]  MomentsOfInertiaUnits=kg*mm^2  ProductsOfInertia=[0 0 0]  ProductsOfInertiaUnits=kg*mm^2  BasedOnType=Density  Density=1000  DensityUnits=kg/(m^3)  DoExposeReferenceFrame=on  SerializedFrames=<Frames/>  GraphicType=FromGeometry  MarkerShape=Sphere  MarkerSize=10  MarkerSizeUnits=m  GraphicVisPropType=SimpleVisualProperties  GraphicDiffuseColor=[0.792156862745098 0.81960784313725488 0.93333333333333335]  GraphicSpecularColor=[0.5 0.5 0.5 1.0]  GraphicAmbientColor=[0.15 0.15 0.15 1.0]  GraphicEmissiveColor=[0.0 0.0 0.0 1.0]  GraphicShininess=75  GraphicOpacity=1  GeometryShape=FromFile  RectangleSize=[1 1]  RectangleSizeUnits=m  BrickDimensions=[1 1 1]  BrickDimensionUnits=m  CylinderRadius=1  CylinderRadiusUnits=m  CylinderLength=1  CylinderLengthUnits=m  SphereRadius=1  SphereRadiusUnits=m  EllipsoidRadii=[1 1 1]  EllipsoidRadiiUnits=m  ExtrusionCrossSection=[1 1; -1 1; -1 -1; 1 -1]  ExtrusionCrossSectionUnits=m  ExtrusionLength=1  ExtrusionLengthUnits=m  PolygonNumSides=3  PolygonOuterRadius=1  PolygonOuterRadiusUnits=m  ExtGeomFileType=STL  ExtGeomFileName=\STL\MOTEUR_Défaut_sldprt.STL  ExtGeomFileUnits=mm  RevolutionCrossSection=[1 1; 1 -1; 2 -1; 2 1]  RevolutionCrossSectionUnits=m  RevolutionExtent=Full  RevolutionAngle=180  RevolutionAngleUnits=deg
  F : PMIOPort  Side=Left
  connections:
  Solid/RConn1 -- ReferenceFrame/RConn1 -- F/RConn1

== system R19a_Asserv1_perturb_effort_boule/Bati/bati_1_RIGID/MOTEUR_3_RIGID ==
  ReferenceFrame : sm_lib/Frames and Transforms/Reference Frame
  Solid : sm_lib/Body Elements/Solid  InertiaType=Custom  Mass=0.064287172119754279  MassUnits=kg  CenterOfMass=[0 32.927342518193171 0]  CenterOfMassUnits=mm  MomentsOfInertia=[23.361167142247837 11.499741081133124 23.353822804254591]  MomentsOfInertiaUnits=kg*mm^2  ProductsOfInertia=[0 0 0]  ProductsOfInertiaUnits=kg*mm^2  BasedOnType=Density  Density=1000  DensityUnits=kg/(m^3)  DoExposeReferenceFrame=on  SerializedFrames=<Frames/>  GraphicType=FromGeometry  MarkerShape=Sphere  MarkerSize=10  MarkerSizeUnits=m  GraphicVisPropType=SimpleVisualProperties  GraphicDiffuseColor=[0.792156862745098 0.81960784313725488 0.93333333333333335]  GraphicSpecularColor=[0.5 0.5 0.5 1.0]  GraphicAmbientColor=[0.15 0.15 0.15 1.0]  GraphicEmissiveColor=[0.0 0.0 0.0 1.0]  GraphicShininess=75  GraphicOpacity=1  GeometryShape=FromFile  RectangleSize=[1 1]  RectangleSizeUnits=m  BrickDimensions=[1 1 1]  BrickDimensionUnits=m  CylinderRadius=1  CylinderRadiusUnits=m  CylinderLength=1  CylinderLengthUnits=m  SphereRadius=1  SphereRadiusUnits=m  EllipsoidRadii=[1 1 1]  EllipsoidRadiiUnits=m  ExtrusionCrossSection=[1 1; -1 1; -1 -1; 1 -1]  ExtrusionCrossSectionUnits=m  ExtrusionLength=1  ExtrusionLengthUnits=m  PolygonNumSides=3  PolygonOuterRadius=1  PolygonOuterRadiusUnits=m  ExtGeomFileType=STL  ExtGeomFileName=\STL\MOTEUR_Défaut_sldprt.STL  ExtGeomFileUnits=mm  RevolutionCrossSection=[1 1; 1 -1; 2 -1; 2 1]  RevolutionCrossSectionUnits=m  RevolutionExtent=Full  RevolutionAngle=180  RevolutionAngleUnits=deg
  F : PMIOPort  Side=Left
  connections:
  Solid/RConn1 -- ReferenceFrame/RConn1 -- F/RConn1

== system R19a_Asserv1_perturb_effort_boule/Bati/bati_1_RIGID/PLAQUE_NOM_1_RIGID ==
  ReferenceFrame : sm_lib/Frames and Transforms/Reference Frame
  Solid : sm_lib/Body Elements/Solid  InertiaType=Custom  Mass=0.00027200040900533893  MassUnits=kg  CenterOfMass=[-0.0026353545106053435 115.22134035146432 0.049293923597036424]  CenterOfMassUnits=mm  MomentsOfInertia=[0.063569474995042688 0.063782951879047547 0.12735197367307241]  MomentsOfInertiaUnits=kg*mm^2  ProductsOfInertia=[2.9045793709905346e-07 6.1711886469806189e-08 2.2164861893284939e-05]  ProductsOfInertiaUnits=kg*mm^2  BasedOnType=Density  Density=1000  DensityUnits=kg/(m^3)  DoExposeReferenceFrame=on  SerializedFrames=<Frames/>  GraphicType=FromGeometry  MarkerShape=Sphere  MarkerSize=10  MarkerSizeUnits=m  GraphicVisPropType=SimpleVisualProperties  GraphicDiffuseColor=[1.0 1.0 1.0]  GraphicSpecularColor=[0.5 0.5 0.5 1.0]  GraphicAmbientColor=[0.15 0.15 0.15 1.0]  GraphicEmissiveColor=[0.0 0.0 0.0 1.0]  GraphicShininess=75  GraphicOpacity=1  GeometryShape=FromFile  RectangleSize=[1 1]  RectangleSizeUnits=m  BrickDimensions=[1 1 1]  BrickDimensionUnits=m  CylinderRadius=1  CylinderRadiusUnits=m  CylinderLength=1  CylinderLengthUnits=m  SphereRadius=1  SphereRadiusUnits=m  EllipsoidRadii=[1 1 1]  EllipsoidRadiiUnits=m  ExtrusionCrossSection=[1 1; -1 1; -1 -1; 1 -1]  ExtrusionCrossSectionUnits=m  ExtrusionLength=1  ExtrusionLengthUnits=m  PolygonNumSides=3  PolygonOuterRadius=1  PolygonOuterRadiusUnits=m  ExtGeomFileType=STL  ExtGeomFileName=\STL\plaque nom simple-1.STL  ExtGeomFileUnits=mm  RevolutionCrossSection=[1 1; 1 -1; 2 -1; 2 1]  RevolutionCrossSectionUnits=m  RevolutionExtent=Full  RevolutionAngle=180  RevolutionAngleUnits=deg
  F : PMIOPort  Side=Left
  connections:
  Solid/RConn1 -- ReferenceFrame/RConn1 -- F/RConn1

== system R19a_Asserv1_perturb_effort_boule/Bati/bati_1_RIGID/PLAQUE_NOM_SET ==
  ReferenceFrame : sm_lib/Frames and Transforms/Reference Frame
  Solid : sm_lib/Body Elements/Solid  InertiaType=Custom  Mass=0.00027200040900533893  MassUnits=kg  CenterOfMass=[-0.0026353545106053435 115.22134035146432 0.049293923597036424]  CenterOfMassUnits=mm  MomentsOfInertia=[0.063569474995042688 0.063782951879047547 0.12735197367307241]  MomentsOfInertiaUnits=kg*mm^2  ProductsOfInertia=[2.9045793709905346e-07 6.1711886469806189e-08 2.2164861893284939e-05]  ProductsOfInertiaUnits=kg*mm^2  BasedOnType=Density  Density=1000  DensityUnits=kg/(m^3)  DoExposeReferenceFrame=on  SerializedFrames=<Frames/>  GraphicType=FromGeometry  MarkerShape=Sphere  MarkerSize=10  MarkerSizeUnits=m  GraphicVisPropType=SimpleVisualProperties  GraphicDiffuseColor=[0.2 0.2 1.0]  GraphicSpecularColor=[0.5 0.5 0.5 1.0]  GraphicAmbientColor=[0.15 0.15 0.15 1.0]  GraphicEmissiveColor=[0.0 0.0 0.0 1.0]  GraphicShininess=75  GraphicOpacity=1  GeometryShape=FromFile  RectangleSize=[1 1]  RectangleSizeUnits=m  BrickDimensions=[1 1 1]  BrickDimensionUnits=m  CylinderRadius=1  CylinderRadiusUnits=m  CylinderLength=1  CylinderLengthUnits=m  SphereRadius=1  SphereRadiusUnits=m  EllipsoidRadii=[1 1 1]  EllipsoidRadiiUnits=m  ExtrusionCrossSection=[1 1; -1 1; -1 -1; 1 -1]  ExtrusionCrossSectionUnits=m  ExtrusionLength=1  ExtrusionLengthUnits=m  PolygonNumSides=3  PolygonOuterRadius=1  PolygonOuterRadiusUnits=m  ExtGeomFileType=STL  ExtGeomFileName=\STL\plaque nom set-1.STL  ExtGeomFileUnits=mm  RevolutionCrossSection=[1 1; 1 -1; 2 -1; 2 1]  RevolutionCrossSectionUnits=m  RevolutionExtent=Full  RevolutionAngle=180  RevolutionAngleUnits=deg
  F : PMIOPort  Side=Left
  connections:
  F/RConn1 -- ReferenceFrame/RConn1 -- Solid/RConn1

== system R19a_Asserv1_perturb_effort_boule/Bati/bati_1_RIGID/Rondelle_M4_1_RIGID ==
  ReferenceFrame : sm_lib/Frames and Transforms/Reference Frame
  Solid : sm_lib/Body Elements/Solid  InertiaType=Custom  Mass=4.0840704496667297e-05  MassUnits=kg  CenterOfMass=[0 0.39999999999999991 0]  CenterOfMassUnits=mm  MomentsOfInertia=[0.00024977494191753434 0.00049519354202209084 0.00024977494191753439]  MomentsOfInertiaUnits=kg*mm^2  ProductsOfInertia=[0 0 0]  ProductsOfInertiaUnits=kg*mm^2  BasedOnType=Density  Density=1000  DensityUnits=kg/(m^3)  DoExposeReferenceFrame=on  SerializedFrames=<Frames/>  GraphicType=FromGeometry  MarkerShape=Sphere  MarkerSize=10  MarkerSizeUnits=m  GraphicVisPropType=SimpleVisualProperties  GraphicDiffuseColor=[0.792156862745098 0.81960784313725488 0.93333333333333335]  GraphicSpecularColor=[0.5 0.5 0.5 1.0]  GraphicAmbientColor=[0.15 0.15 0.15 1.0]  GraphicEmissiveColor=[0.0 0.0 0.0 1.0]  GraphicShininess=75  GraphicOpacity=1  GeometryShape=FromFile  RectangleSize=[1 1]  RectangleSizeUnits=m  BrickDimensions=[1 1 1]  BrickDimensionUnits=m  CylinderRadius=1  CylinderRadiusUnits=m  CylinderLength=1  CylinderLengthUnits=m  SphereRadius=1  SphereRadiusUnits=m  EllipsoidRadii=[1 1 1]  EllipsoidRadiiUnits=m  ExtrusionCrossSection=[1 1; -1 1; -1 -1; 1 -1]  ExtrusionCrossSectionUnits=m  ExtrusionLength=1  ExtrusionLengthUnits=m  PolygonNumSides=3  PolygonOuterRadius=1  PolygonOuterRadiusUnits=m  ExtGeomFileType=STL  ExtGeomFileName=\STL\Rondelle M4_Défaut_sldprt.STL  ExtGeomFileUnits=mm  RevolutionCrossSection=[1 1; 1 -1; 2 -1; 2 1]  RevolutionCrossSectionUnits=m  RevolutionExtent=Full  RevolutionAngle=180  RevolutionAngleUnits=deg
  F : PMIOPort  Side=Left
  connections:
  Solid/RConn1 -- ReferenceFrame/RConn1 -- F/RConn1

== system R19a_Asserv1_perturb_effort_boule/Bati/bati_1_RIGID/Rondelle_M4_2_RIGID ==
  ReferenceFrame : sm_lib/Frames and Transforms/Reference Frame
  Solid : sm_lib/Body Elements/Solid  InertiaType=Custom  Mass=4.0840704496667297e-05  MassUnits=kg  CenterOfMass=[0 0.39999999999999991 0]  CenterOfMassUnits=mm  MomentsOfInertia=[0.00024977494191753434 0.00049519354202209084 0.00024977494191753439]  MomentsOfInertiaUnits=kg*mm^2  ProductsOfInertia=[0 0 0]  ProductsOfInertiaUnits=kg*mm^2  BasedOnType=Density  Density=1000  DensityUnits=kg/(m^3)  DoExposeReferenceFrame=on  SerializedFrames=<Frames/>  GraphicType=FromGeometry  MarkerShape=Sphere  MarkerSize=10  MarkerSizeUnits=m  GraphicVisPropType=SimpleVisualProperties  GraphicDiffuseColor=[0.792156862745098 0.81960784313725488 0.93333333333333335]  GraphicSpecularColor=[0.5 0.5 0.5 1.0]  GraphicAmbientColor=[0.15 0.15 0.15 1.0]  GraphicEmissiveColor=[0.0 0.0 0.0 1.0]  GraphicShininess=75  GraphicOpacity=1  GeometryShape=FromFile  RectangleSize=[1 1]  RectangleSizeUnits=m  BrickDimensions=[1 1 1]  BrickDimensionUnits=m  CylinderRadius=1  CylinderRadiusUnits=m  CylinderLength=1  CylinderLengthUnits=m  SphereRadius=1  SphereRadiusUnits=m  EllipsoidRadii=[1 1 1]  EllipsoidRadiiUnits=m  ExtrusionCrossSection=[1 1; -1 1; -1 -1; 1 -1]  ExtrusionCrossSectionUnits=m  ExtrusionLength=1  ExtrusionLengthUnits=m  PolygonNumSides=3  PolygonOuterRadius=1  PolygonOuterRadiusUnits=m  ExtGeomFileType=STL  ExtGeomFileName=\STL\Rondelle M4_Défaut_sldprt.STL  ExtGeomFileUnits=mm  RevolutionCrossSection=[1 1; 1 -1; 2 -1; 2 1]  RevolutionCrossSectionUnits=m  RevolutionExtent=Full  RevolutionAngle=180  RevolutionAngleUnits=deg
  F : PMIOPort  Side=Left
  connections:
  Solid/RConn1 -- ReferenceFrame/RConn1 -- F/RConn1

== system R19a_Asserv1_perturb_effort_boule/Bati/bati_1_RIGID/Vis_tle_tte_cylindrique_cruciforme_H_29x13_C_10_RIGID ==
  ReferenceFrame : sm_lib/Frames and Transforms/Reference Frame
  Solid : sm_lib/Body Elements/Solid  InertiaType=Custom  Mass=8.3821869835456372e-05  MassUnits=kg  CenterOfMass=[4.9478681581074904 0.00064910481891303923 -0.0013634218224953438]  CenterOfMassUnits=mm  MomentsOfInertia=[0.00016543197172893975 0.0014334630955093895 0.0014333390308476422]  MomentsOfInertiaUnits=kg*mm^2  ProductsOfInertia=[-5.4062904633677868e-09 -1.3111174919527308e-07 6.0713893531177014e-07]  ProductsOfInertiaUnits=kg*mm^2  BasedOnType=Density  Density=1000  DensityUnits=kg/(m^3)  DoExposeReferenceFrame=on  SerializedFrames=<Frames/>  GraphicType=FromGeometry  MarkerShape=Sphere  MarkerSize=10  MarkerSizeUnits=m  GraphicVisPropType=SimpleVisualProperties  GraphicDiffuseColor=[0.75294117647058822 0.75294117647058822 0.75294117647058822]  GraphicSpecularColor=[0.5 0.5 0.5 1.0]  GraphicAmbientColor=[0.15 0.15 0.15 1.0]  GraphicEmissiveColor=[0.0 0.0 0.0 1.0]  GraphicShininess=75  GraphicOpacity=1  GeometryShape=FromFile  RectangleSize=[1 1]  RectangleSizeUnits=m  BrickDimensions=[1 1 1]  BrickDimensionUnits=m  CylinderRadius=1  CylinderRadiusUnits=m  CylinderLength=1  CylinderLengthUnits=m  SphereRadius=1  SphereRadiusUnits=m  EllipsoidRadii=[1 1 1]  EllipsoidRadiiUnits=m  ExtrusionCrossSection=[1 1; -1 1; -1 -1; 1 -1]  ExtrusionCrossSectionUnits=m  ExtrusionLength=1  ExtrusionLengthUnits=m  PolygonNumSides=3  PolygonOuterRadius=1  PolygonOuterRadiusUnits=m  ExtGeomFileType=STL  ExtGeomFileName=\STL\Vis à tôle tête cylindrique cruciforme H 2-9x13 - C_Réaliste_sldprt.STL  ExtGeomFileUnits=mm  RevolutionCrossSection=[1 1; 1 -1; 2 -1; 2 1]  RevolutionCrossSectionUnits=m  RevolutionExtent=Full  RevolutionAngle=180  RevolutionAngleUnits=deg
  F : PMIOPort  Side=Left
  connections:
  Solid/RConn1 -- ReferenceFrame/RConn1 -- F/RConn1
